|Texas Instruments Incorporated
| "SMART" 4-Wire Touch Screen Controller with Stereo DAC / Mono ADC
| with HP/Speaker Amplifier
| Marketing part#   Digital Voltage Range   Package-type   #pins
| TSC2100IDA   1.1V - 3.6V   TSSOP   32
| TSC2100IDAG4   1.1V - 3.6V   TSSOP   32
| TSC2100IRHB   1.1V - 3.6V   QFN   32
| TSC2100IRHBG4   1.1V - 3.6V   QFN   32
| TSC2100IRHBR   1.1V - 3.6V   QFN   32
| TSC2100IRHBRG4   1.1V - 3.6V   QFN   32
[IBIS Ver]   3.2
[File name]   tsc2100.ibs
|SIMDE Ver   V3.0 - 201101 - RHL4 - Build 457
[File Rev]   1.1
[Date]   9/15/2011
[Source]
| Texas Instruments Incorporated.
| Analog-eLab Design Center, HPA
| 12500 TI Blvd
| Dallas, TX -75243
| e-mail: elab_scm_ibis@list.ti.com
[Notes]   Revision History:
| Rev 1.1: 9/15/2011
| - Updated C_comp values without Bondpad.
| Rev 1.0: 8/24/2011
| - Initial version of the model
| - Model generated from simulations in TISPICE
| - Model matched to SPICE simulation
| - C_comp although listed in numerical order of value are
|   obtained from varying PVT conditions. For PVT conditions for
|   each specific value refer the buffer description under
|   respective [Model]. IBIS model user is responsible for using
|   appropriate C_comp to simulate for Signal Integrity.
| - Model names with a trailing _1p8 contains the model for
|   1.8V [1.62V and 1.98V].Model names with a trailing _3p3
|   contains the model for 3.3V [3.0V and 3.6V].
[Disclaimer]
| This model is designed as an aid for customers of Texas Instruments.
| TI and its licensors and suppliers make no warranties, either expressed
| or implied, with respect to this  model, including the warranties of
| merchantability or fitness for a particular purpose. The model is
| provided solely on an "as is" basis. The entire risk as to its quality
| and performance is with the customer.
[Copyright]
 (C) Copyright 2011 Texas Instruments Incorporated.All rights reserved.
|   TSC2100DA
[Component]   TSC2100DA
[Manufacturer]   TI
[Package]   |32 TSSOP   -  DA package
|   typ   min   max
R_pkg   0.20750   0.15801   0.27289
L_pkg   3.38285nH   2.40689nH   5.01067nH
C_pkg   0.79971pF   0.66567pF   0.94217pF
[Pin]  signal_name   model_name   R_pin   L_pin   C_pin
1   DIN   INPUT   0.26799   4.84342nH  0.93124pF
2   DOUT   OUTPUT   0.23712   4.07645nH  0.87884pF
3   BCLK   IO   0.21588   3.32515nH  0.80860pF
4   DVDD   POWER   0.15667   2.55370nH  0.84193pF
5   DVSS   GND   0.14312   2.41927nH  0.80709pF
6   IOVDD   POWER   0.13500   2.38539nH  0.73509pF
7   MCLK   INPUT   0.16852   2.52375nH  0.69134pF
8   SCLK   INPUT   0.15877   2.41392nH  0.67038pF
9   MISO   OUTPUT   0.15938   2.42311nH  0.69009pF
10   MOSI   INPUT   0.16666   2.50863nH  0.68612pF
11   _SS   INPUT   0.17706   2.63272nH  0.71660pF
12   _PINTDAV   OUTPUT   0.19201   2.82730nH  0.77774pF
13   MICBIAS   TERM   0.19984   2.95712nH  0.79014pF
14   MICIN   TERM   0.21155   3.26724nH  0.80378pF
15   AUX   TERM   0.24310   4.20222nH  0.88443pF
16   VBAT2   TERM   0.26991   4.90180nH  0.93381pF
17   VBAT1   TERM   0.26263   4.81995nH  0.93120pF
18   VREF   TERM   0.23242   4.05017nH  0.88009pF
19   AVSS   GND   0.15019   2.79631nH  0.85162pF
20   Y-   TERM   0.19482   2.96952nH  0.79400pF
21   X-   TERM   0.18396   2.75027nH  0.77804pF
22   Y+   TERM   0.17374   2.60830nH  0.71764pF
23   X+   TERM   0.16588   2.49631nH  0.68584pF
24   AVDD   POWER   0.11707   2.19794nH  0.69634pF
25   HPL   TERM   0.15801   2.40689nH  0.66567pF
26   DRVSS   GND   0.12264   2.26194nH  0.73108pF
27   VGND   GND   0.13246   2.42360nH  0.76410pF
28   DRVDD   POWER   0.14317   2.58784nH  0.82922pF
29   HPR   TERM   0.20226   3.17746nH  0.76570pF
30   _RESET   INPUT   0.22150   3.69611nH  0.85134pF
31   LRCK   IO   0.24293   4.29987nH  0.91823pF
32   _PWD/ADWS   IO   0.27289   5.01067nH  0.94217pF
33   THERMAL_PAD   NC   0.00008   0.00125nH  3.26032pF
[Pin Mapping]  pulldown_ref pullup_ref gnd_clamp_ref power_clamp_ref
1   GNDBUS3   PWRBUS2
2   GNDBUS1   PWRBUS2
3   GNDBUS1   PWRBUS2
4   NC   PWRBUS1
5   GNDBUS1   NC
6   NC   PWRBUS2
7   GNDBUS3   PWRBUS2
8   GNDBUS3   PWRBUS2
9   GNDBUS1   PWRBUS2
10   GNDBUS3   PWRBUS2
11   GNDBUS3   PWRBUS2
12   GNDBUS1   PWRBUS2
13   GNDBUS3   PWRBUS3
14   GNDBUS3   PWRBUS3
15   GNDBUS3   NC
16   GNDBUS3   PWRBUS3
17   GNDBUS3   PWRBUS3
18   GNDBUS3   PWRBUS3
19   GNDBUS2   NC
20   GNDBUS3   NC
21   GNDBUS3   NC
22   GNDBUS3   NC
23   GNDBUS3   NC
24   NC   PWRBUS3
25   GNDBUS3   PWRBUS4
26   GNDBUS3   NC
27   GNDBUS4   NC
28   NC   PWRBUS4
29   GNDBUS3   PWRBUS4
30   GNDBUS3   PWRBUS2
31   GNDBUS1   PWRBUS2
32   GNDBUS1   PWRBUS2
33   NC   NC
|   TSC2100RHB
[Component]   TSC2100RHB
[Manufacturer]   TI
[Package]   |32 QFN   -  RHB package
|   typ   min   max
R_pkg   0.10351   0.08210   0.12918
L_pkg   1.61625nH   1.24160nH   2.06878nH
C_pkg   0.14271pF   0.12253pF   0.15971pF
[Pin]  signal_name   model_name   R_pin   L_pin   C_pin
1   DVSS   GND   0.05924   1.55564nH  0.18377pF
2   IOVDD   POWER   0.05859   1.52995nH  0.18507pF
3   MCLK   INPUT   0.11553   1.82190nH  0.15746pF
4   SCLK   INPUT   0.11037   1.73300nH  0.15617pF
5   MISO   OUTPUT   0.11080   1.74171nH  0.15337pF
6   MOSI   INPUT   0.11477   1.81191nH  0.15333pF
7   _SS   INPUT   0.11934   1.89293nH  0.15971pF
8   _PINTDAV   OUTPUT   0.12918   2.06878nH  0.15831pF
9   MICBIAS   TERM   0.10633   1.66917nH  0.13890pF
10   MICIN   TERM   0.09288   1.43384nH  0.13421pF
11   AUX   TERM   0.09150   1.40990nH  0.13130pF
12   VBAT2   TERM   0.08318   1.26720nH  0.12276pF
13   VBAT1   TERM   0.08210   1.24900nH  0.12270pF
14   VREF   TERM   0.08477   1.29460nH  0.12718pF
15   AVSS   GND   0.04630   1.04858nH  0.17539pF
16   Y-   TERM   0.11299   1.78598nH  0.14855pF
17   X-   TERM   0.12361   1.97037nH  0.15592pF
18   Y+   TERM   0.11565   1.82774nH  0.15719pF
19   X+   TERM   0.11212   1.76480nH  0.15295pF
20   AVDD   POWER   0.05515   1.40936nH  0.18050pF
21   HPL   TERM   0.10998   1.72630nH  0.15269pF
22   DRVSS   GND   0.05682   1.46085nH  0.20489pF
23   VGND   GND   0.06033   1.58220nH  0.21951pF
24   DRVDD   POWER   0.06540   1.76550nH  0.21225pF
25   HPR   TERM   0.12916   2.06107nH  0.15686pF
26   _RESET   INPUT   0.10172   1.57994nH  0.13922pF
27   LRCK   IO   0.09080   1.38990nH  0.13251pF
28   _PWD/ADWS   IO   0.08402   1.27310nH  0.12381pF
29   DIN   INPUT   0.08219   1.24160nH  0.12253pF
30   DOUT   OUTPUT   0.08610   1.30890nH  0.12835pF
31   BCLK   IO   0.09519   1.46643nH  0.13894pF
32   DVDD   POWER   0.05399   1.23260nH  0.19255pF
[Pin Mapping]  pulldown_ref pullup_ref gnd_clamp_ref power_clamp_ref
1   GNDBUS1   NC
2   NC   PWRBUS2
3   GNDBUS3   PWRBUS2
4   GNDBUS3   PWRBUS2
5   GNDBUS1   PWRBUS2
6   GNDBUS3   PWRBUS2
7   GNDBUS3   PWRBUS2
8   GNDBUS1   PWRBUS2
9   GNDBUS3   PWRBUS3
10   GNDBUS3   PWRBUS3
11   GNDBUS3   NC
12   GNDBUS3   PWRBUS3
13   GNDBUS3   PWRBUS3
14   GNDBUS3   PWRBUS3
15   GNDBUS2   NC
16   GNDBUS3   NC
17   GNDBUS3   NC
18   GNDBUS3   NC
19   GNDBUS3   NC
20   NC   PWRBUS3
21   GNDBUS3   PWRBUS4
22   GNDBUS3   NC
23   GNDBUS4   NC
24   NC   PWRBUS4
25   GNDBUS3   PWRBUS4
26   GNDBUS3   PWRBUS2
27   GNDBUS1   PWRBUS2
28   GNDBUS1   PWRBUS2
29   GNDBUS3   PWRBUS2
30   GNDBUS1   PWRBUS2
31   GNDBUS1   PWRBUS2
32   NC   PWRBUS1
|   Model Selectors
[Model Selector] INPUT
input_1p8  1.8V digital input
input_3p3  3.3V digital input
[Model Selector] OUTPUT
output_1p8  1.8V digital output
output_3p3  3.3V digital output
[Model Selector] IO
io_1p8  1.8V digital I/O
io_3p3  3.3V digital I/O
[Model Selector] TERM
term_1-8V  1.8V nominal termination
term_3-3V  3.3V nominal termination
[Model] term_1-8V
Model_type Terminator
C_comp   1.0e-20F  1.0e-20F  1.0e-20F
|   typ   min   max
[Voltage Range]   1.8V   1.62V   1.98V
[POWER Clamp Reference]   1.8V   1.62V   1.98V
[GND Clamp Reference]   0V   0V   0V
|Ambient Temperature   25   85   -40
|Junction Temperature
[Temperature Range]   26   86   -40
[Model] term_3-3V
Model_type Terminator
C_comp   1.0e-20F  1.0e-20F  1.0e-20F
|   typ   min   max
[Voltage Range]   3.3V   3.0V   3.6V
[POWER Clamp Reference]   3.3V   3.0V   3.6V
[GND Clamp Reference]   0V   0V   0V
|Ambient Temperature   25   85   -40
|Junction Temperature
[Temperature Range]   26   86   -40
| Models and submodels in the file (8): input_1p8 (Input), input_3p3 (Input), output_1p8 (Output), output_3p3 (Output), io_1p8 (I/O), io_3p3 (I/O), term_1-8V (Terminator), term_3-3V (Terminator)
